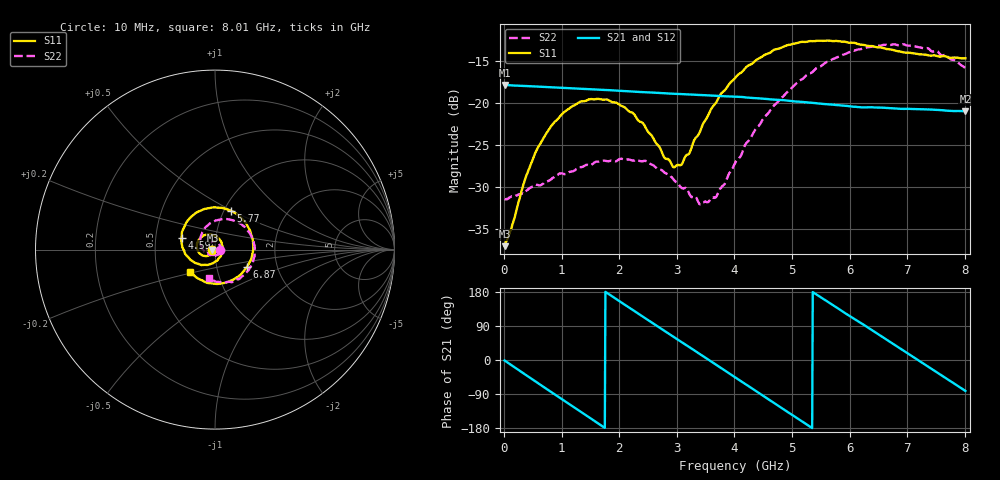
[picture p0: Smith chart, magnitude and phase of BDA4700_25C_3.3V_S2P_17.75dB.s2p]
!Agilent Technologies,E5071B,MY42404982,A.09.10
!Date: Mon Oct 20 18:10:29 2025
!Data & Calibration Information:
!Freq	S11:SOLT2(ON)	S21:SOLT2(ON)	S12:SOLT2(ON)	S22:SOLT2(ON)
# Hz S RI R 50
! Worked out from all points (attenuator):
!   801 points, 10 MHz to 8.01 GHz, reference 50 ohm
!   highest |S21| = -17.84 dB at 10 MHz (marker M1); lowest = -21.0 dB at 8.01 GHz (marker M2)
!   lowest |S11| = -37.0 dB at 10 MHz (marker M3), VSWR 1.03, Z = 48.6 - j0.137 ohm
!   |S11| at or under -10 dB: start of sweep to end of sweep
!   |S22| runs from -32.1 to -13.0 dB; largest |S21 - S12| = 0.0015
!   S11 on the Smith chart (normalised r, x): 10 MHz: 0.97, -0.00; 4.59 GHz: 0.68, +0.09; 5.77 GHz: 1.07, +0.49; 6.87 GHz: 1.40, -0.28; 8.01 GHz: 0.74, -0.19
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1e7  -0.014 -0.00141  0.1282 -0.00281  0.1281 -0.00288  0.0268 -0.000872
3.7e8  -0.0244 -0.0258  0.0988 -0.0787  0.0987 -0.0787  0.0221 -0.0196
5.8e8  -0.0406 -0.0351  0.0624 -0.1086  0.0624 -0.1086  0.0143 -0.0293
1e9  -0.0818 -0.0246  -0.0278 -0.1201  -0.0278 -0.1203  -0.0153 -0.035
1.35e9  -0.1017 0.0115  -0.0913 -0.0804  -0.0913 -0.0805  -0.0377 -0.0175
2.07e9  -0.0443 0.0843  -0.1006 0.0615  -0.1007 0.0616  -0.0294 0.0357
2.68e9  0.0346 0.0436  0.00522 0.1148  0.00498 0.1147  0.0161 0.0371
2.93e9  0.0417 0.00341  0.0525 0.1008  0.0524 0.1006  0.0272 0.0226
3.07e9  0.0375 -0.0205  0.0752 0.0845  0.0744 0.085  0.0295 0.0112
3.4e9  -4.7e-05 -0.0672  0.1075 0.0302  0.1076 0.0302  0.021 -0.0135
3.54e9  -0.0249 -0.0801  0.111 0.00326  0.1111 0.00307  0.0123 -0.0226
3.69e9  -0.0561 -0.0849  0.1074 -0.0253  0.1075 -0.0257  -0.001 -0.0279
4.01e9  -0.1248 -0.0649  0.0766 -0.0778  0.0767 -0.0775  -0.0344 -0.0269
4.59e9  -0.1862 0.0648  -0.0252 -0.1025  -0.0249 -0.1026  -0.0801 0.0347
4.94e9  -0.1533 0.1601  -0.0776 -0.068  -0.0774 -0.0686  -0.0719 0.0939
5.35e9  -0.048 0.2285  -0.1003 -0.000573  -0.1003 -0.00116  -0.0141 0.1518
5.77e9  0.0872 0.2171  -0.0734 0.064  -0.0731 0.0641  0.0814 0.1672
6.24e9  0.1944 0.1072  -0.00562 0.0941  -0.00417 0.0942  0.1836 0.1042
6.68e9  0.2053 -0.0383  0.0602 0.0713  0.0604 0.0713  0.2208 -0.0067
6.87e9  0.1784 -0.0962  0.079 0.0482  0.0792 0.0475  0.2129 -0.0609
7.45e9  0.0179 -0.1914  0.082 -0.04  0.082 -0.0402  0.1054 -0.1725
8.01e9  -0.1386 -0.1221  0.0128 -0.0883  0.0132 -0.0885  -0.0355 -0.1574
